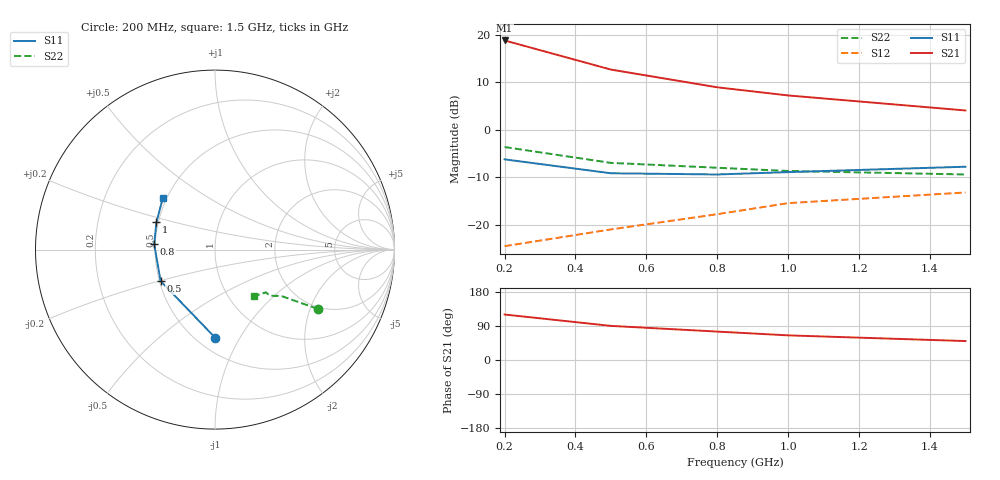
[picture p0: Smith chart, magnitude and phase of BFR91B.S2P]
! SCCS file tdata/motorola: @(#)get -r1.1 /eesof/src/tdata/motorola/s.bfr91b.s2p # Version date: 10/22/90
!  BFR91B.S2P
!  BFR91
!  VCE=5V; IC=5mA
#  GHZ S MA R 50
!  S-PARAMETER DATA
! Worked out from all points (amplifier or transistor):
!   5 points, 200 MHz to 1.5 GHz, reference 50 ohm
!   highest |S21| = 18.8 dB at 200 MHz (marker M1)
!   |S21| within 3 dB of that: start of sweep to 347 MHz
!   unconditionally stable (mu >= 1): 618.1 MHz to end of sweep
!   at 200 MHz: K = 0.54, MSG = 21.6 dB, |S12| = -24.4 dB
!   at 800 MHz: K = 1.07, MAG = 11.8 dB, |S12| = -17.7 dB
!   at 1.5 GHz: K = 1.10, MAG = 6.7 dB, |S12| = -13.2 dB
!   S11 on the Smith chart (normalised r, x): 200 MHz: 0.61, -0.79; 500 MHz: 0.51, -0.20; 800 MHz: 0.49, +0.03; 1 GHz: 0.49, +0.17; 1.5 GHz: 0.48, +0.33
0.2  0.49 -90.0  8.7 120.0  0.06 55.0  0.66 -30.0
0.5  0.35 -150.0  4.3 90.0  0.09 60.0  0.45 -35.0
0.8  0.34 175.0  2.8 75.0  0.13 65.0  0.4 -40.0
1  0.36 155.0  2.3 65.0  0.17 65.0  0.37 -40.0
1.5  0.41 135.0  1.6 50.0  0.22 65.0  0.34 -50.0
